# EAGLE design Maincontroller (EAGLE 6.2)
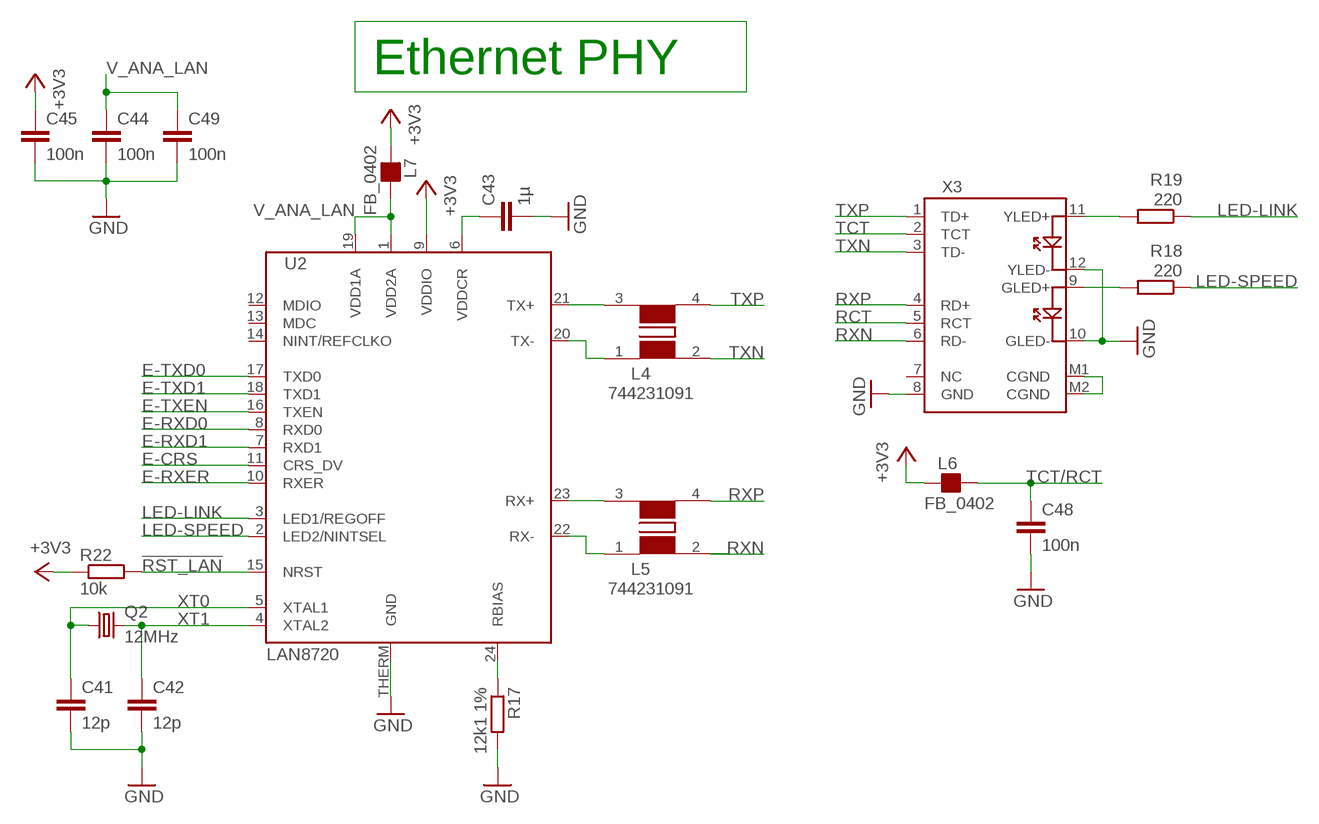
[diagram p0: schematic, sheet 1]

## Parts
C41  12p  C-EUC0402  [C0402]
C42  12p  C-EUC0402  [C0402]
C43  1µ  C-EUC0402  [C0402]
C44  100n  C-EUC0402  [C0402]
C45  100n  C-EUC0402  [C0402]
C48  100n  C-EUC0402  [C0402]
C49  100n  C-EUC0402  [C0402]
L4  744231091  WE-CNS_0805  [WE-CNS_0805]
L5  744231091  WE-CNS_0805  [WE-CNS_0805]
L6  FB_0402  [L0402]
L7  FB_0402  [L0402]
Q2  12MHz  CRYSTALHC49U-V  [HC49U-V]
R17  12k1 1%  R-EU_R0402  [R0402]
R18  220  R-EU_R0402  [R0402]
R19  220  R-EU_R0402  [R0402]
R22  10k  R-EU_R0402  [R0402]
U2  LAN8720  [QFN24_4MM]
X3  MAGJACK  [MAGJACK]

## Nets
!RST_LAN: R22.2 U2.15(NRST)
+3V3: C45.1 L6.1 L7.1 R22.1 U2.9(VDDIO)
E-CRS: U2.11(CRS_DV)
E-RXD0: U2.8(RXD0)
E-RXD1: U2.7(RXD1)
E-RXER: U2.10(RXER)
E-TXD0: U2.17(TXD0)
E-TXD1: U2.18(TXD1)
E-TXEN: U2.16(TXEN)
GND: C41.2 C42.2 C43.2 C44.2 C45.2 C48.2 C49.2 R17.2 U2.THERM(GND) X3.8(GND) X3.10(GLED-) X3.12(YLED-)
LED-LINK: R19.1 U2.3(LED1/REGOFF)
LED-SPEED: R18.1 U2.2(LED2/NINTSEL)
N$7: X3.M1(CGND) X3.M2(CGND)
N$9: C43.1 U2.6(VDDCR)
N$22: R19.2 X3.11(YLED+)
N$23: R18.2 X3.9(GLED+)
RBIAS: R17.1 U2.24(RBIAS)
RXN: L5.2 X3.6(RD-)
RXN-C: L5.1 U2.22(RX-)
RXP: L5.4 X3.4(RD+)
RXP-C: L5.3 U2.23(RX+)
TCT/RCT: C48.1 L6.2 X3.2(TCT) X3.5(RCT)
TXN: L4.2 X3.3(TD-)
TXN-C: L4.1 U2.20(TX-)
TXP: L4.4 X3.1(TD+)
TXP-C: L4.3 U2.21(TX+)
V_ANA_LAN: C44.1 C49.1 L7.2 U2.1(VDD2A) U2.19(VDD1A)
XT0: C41.1 Q2.1 U2.5(XTAL1)
XT1: C42.1 Q2.2 U2.4(XTAL2)
Unconnected: U2.12(MDIO) U2.13(MDC) U2.14(NINT/REFCLKO)

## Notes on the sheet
- Ethernet PHY
- TCT
- RCT

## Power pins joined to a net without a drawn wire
NC: X3.7(NC)

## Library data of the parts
C41-C45 C48 C49 = _rcl:C-EU: CAPACITOR, European symbol
L4 L5 = wuerth-elektronik:WE-CNS: SMD Multilayer Common-Mode Choke WE-CNS - Common mode data line filter - Fully shielded -- USB 2.0 -- IEEE 1394 -- Power supply systems -- Signal interfaces
L6 L7 = _rc-master-smd:FB_: FERRITE BEAD
Q2 = _crystal:CRYSTAL: CRYSTAL; OC_FARNELL: 1666969; OC_NEWARK: unknown
R17-R19 R22 = _rcl:R-EU_: RESISTOR, European symbol
U2 = _microbuilder:LAN8720: LAN8720A 10/100 Ethernet PHY Mouser: 886-LAN8720AI-CP
X3 = _IT-WNS:MAGJACK: MagJack von IT-WNS Art.Nr: RJ45-TRAFO-L AMPHENOL Connector FROM: "Drawing Nr. LMJ199 882X 110DTLX39J Datasheet: C:\Dokumente und Einstellungen\rene\Eigene Dateien\elektro\datenblätter\IT-WNS ArtNr RJ45-TRAFO-L.pdf

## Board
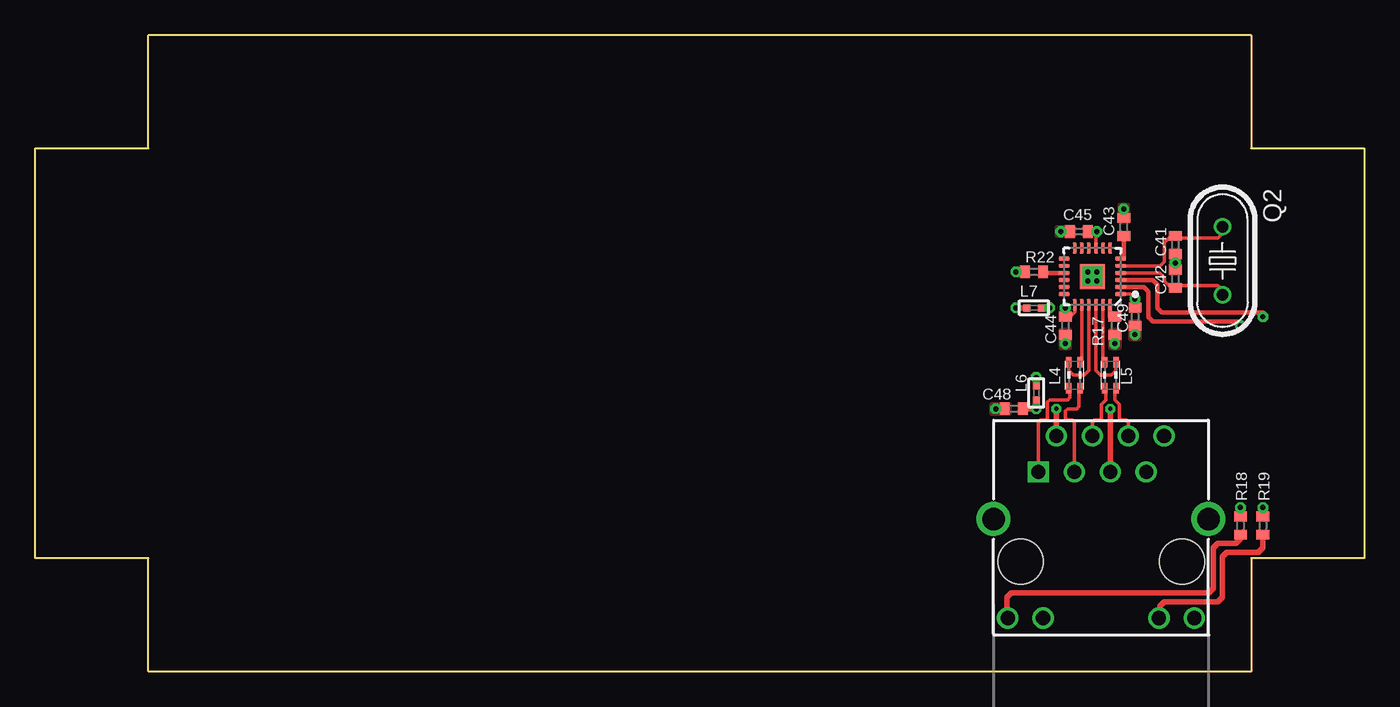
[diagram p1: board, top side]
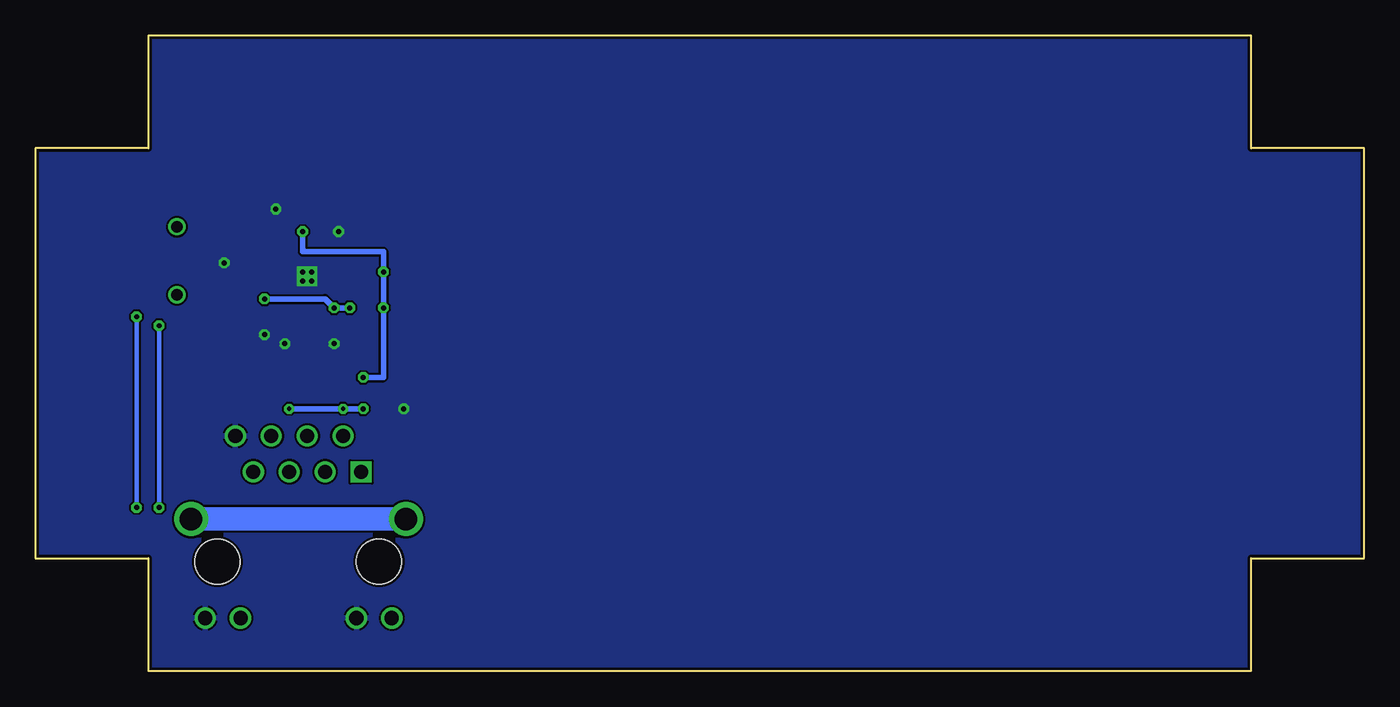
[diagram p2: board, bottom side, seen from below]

Size 94 x 45 mm. Coordinates in mm from the lower left corner, seen from the top.
Copper layers (1*16): Top 0.035mm / dielectric 1.5mm / Bottom 0.035mm
Design rules: minimum track width 0.15mm, minimum drill 0.3mm, track to track 0.15mm, track to pad 0.15mm, pad to pad 0.15mm, via to via 0.15mm, smd to smd 0mil, copper to edge 0.2mm, drill to drill 0.2mm, minimum pad ring 0.2mm, minimum via ring 0.2mm, stop-mask expansion 3mil, vias tented up to drill 0.8mm, thermal gap 0.15mm

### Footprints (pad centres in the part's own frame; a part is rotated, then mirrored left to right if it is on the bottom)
C0402 = smd 0.7 x 0.9: 1 -0.65,0; 2 0.65,0
WE-CNS_0805 = smd 0.75 x 0.4: 1 -0.925,0.4; 2 0.925,0.4; 3 -0.925,-0.4; 4 0.925,-0.4
L0402 = smd 0.5 x 0.5: 1 -0.508,0; 2 0.508,0
HC49U-V = drill 0.813: 1 -2.413,0; 2 2.413,0
R0402 = smd 0.7 x 0.9: 1 -0.65,0; 2 0.65,0
QFN24_4MM = smd 0.8 x 0.28: 1 -2,1.25; 2 -2,0.75; 3 -2,0.25; 4 -2,-0.25; 5 -2,-0.75; 6 -2,-1.25; 13 2,-1.25; 14 2,-0.75; 15 2,-0.25; 16 2,0.25; 17 2,0.75; 18 2,1.25 | smd 0.28 x 0.8: 7 -1.25,-2; 8 -0.75,-2; 9 -0.25,-2; 10 0.25,-2; 11 0.75,-2; 12 1.25,-2; 19 1.25,2; 20 0.75,2; 21 0.25,2; 22 -0.25,2; 23 -0.75,2; 24 -1.25,2 | smd 1.778 x 1.778: THERM 0,0
MAGJACK = drill 1 square: 1 3.175,17.445 | drill 1: 2 4.445,19.985; 3 5.715,17.445; 4 6.985,19.985; 5 8.255,17.445; 6 9.525,19.985; 7 10.795,17.445; 8 12.065,19.985; 9 1,7.1; 10 3.5,7.1; 11 11.7,7.1; 12 14.2,7.1 | drill 1.6: M1 0,14.1; M2 15.2,14.1 | hole 3.2: 1.905,11.095; 13.335,11.095

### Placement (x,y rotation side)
C41  80.64,30.16 270 top
C42  80.64,27.78 90 top
C43  76.99,31.43 90 top
C44  72.87,24.45 270 top
C45  73.82,31.11 180 top
C48  69.22,18.57 180 top
C49  77.79,25.08 270 top
L4  73.5,20.95 270 top
L5  76.04,20.95 270 top
L6  70.8,19.68 270 top
L7  70.64,25.72 0 top
Q2  83.98,29.05 270 top
R17  76.36,24.45 270 top
R18  85.25,10.32 270 top
R19  86.84,10.32 270 top
R22  70.64,28.26 0 top
U2  74.77,27.94 180 top
U$2  [KL_W_GEHÄUSE]  0,0 90 bottom
X3  67.79,-3.33 0 top

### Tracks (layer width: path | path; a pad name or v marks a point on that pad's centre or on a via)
!RST_LAN
  Top 0.305: U2.15 71.29,28.19 R22.2
+3V3  (via drill 0.35)
  Top 0.254: U2.9 75.02,31.11 v75.09,31.11 74.93,31.11
  Top 0.305: C45.1 74.93,31.11 75.02,31.11
  Top 0.406: L6.1 v70.8,20.8 | R22.1 v69.37,28.26 | L7.1 v69.37,25.72
  Bottom 0.406: v70.8,20.8 69.37,20.8 v69.37,25.72 v69.37,28.26 69.37,29.69 75.09,29.69 v75.09,31.11
GND  (via drill 0.35)
  Top 0.305: v75.09,27.62 U2.THERM 74.77,27.62
  other vias: 74.45,28.26 75.09,28.26 74.45,27.62 76.36,23.18 80.64,28.89 76.99,32.7 72.87,23.18 72.55,31.11 67.94,18.57 77.79,23.81
  pour Bottom: 0,45.09 93.98,45.09 93.98,0 0,0
  pour Top (no thermals): 76.68,24.13 76.04,24.13 76.04,22.86 76.68,22.86
  pour Top (no thermals): 76.68,31.75 77.31,31.75 77.31,33.02 76.68,33.02
  pour Top (no thermals): 73.18,24.13 72.55,24.13 72.55,22.86 73.18,22.86
  pour Top (no thermals): 73.5,30.8 73.5,31.43 72.23,31.43 72.23,30.8
  pour Top (no thermals): 67.63,18.89 67.63,18.26 68.9,18.26 68.9,18.89
  pour Top (no thermals): 80.33,28.1 80.96,28.1 80.96,29.84 80.33,29.84
  pour Top (no thermals): 78.11,24.77 77.47,24.77 77.47,23.5 78.11,23.5
LED-LINK  (via drill 0.35)
  Top 0.305: U2.3 79.06,27.69 79.38,27.37 79.38,25.72 79.69,25.4 86.84,25.4 v86.84,25.08 | v86.84,11.59 R19.1
  Bottom 0.305: v86.84,25.08 v86.84,11.59
LED-SPEED  (via drill 0.35)
  Top 0.305: U2.2 78.42,27.19 78.74,26.87 78.74,25.08 79.06,24.77 85.25,24.77 v85.25,24.45 | v85.25,11.59 R18.1
  Bottom 0.305: v85.25,24.45 v85.25,11.59
N$7
  Bottom 1.676: X3.M1 X3.M2
N$9
  Top 0.305: U2.6 76.99,29.19 C43.1
N$22
  Top 0.406: X3.11 79.53,3.77 79.53,4.6 79.85,4.92 83.66,4.92 83.98,5.24 83.98,8.1 84.3,8.41 86.52,8.41 86.84,8.73 R19.2
N$23
  Top 0.406: X3.9 68.74,3.77 68.74,5.24 69.06,5.56 83.03,5.56 83.34,5.87 83.34,8.73 83.66,9.05 84.93,9.05 85.25,9.37 R18.2
RBIAS
  Top 0.305: R17.1 76.02,25.08 U2.24
RXN
  Top 0.254: L5.2 76.36,20.03 76.36,19.21 76.68,18.89 76.68,17.94 76.83,17.78 77.17,17.78 77.33,17.62 77.33,16.65 X3.6
RXN-C
  Top 0.254: L5.1 76.44,21.27 76.12,20.95 75.34,20.95 75.02,21.27 U2.22
RXP
  Top 0.254: L5.4 75.72,20.03 75.72,19.21 75.41,18.89 75.41,17.94 75.25,17.78 74.92,17.78 74.76,17.62 74.76,16.65 X3.4
RXP-C
  Top 0.254: L5.3 75.52,21.88 U2.23
TCT/RCT  (via drill 0.3, 0.35)
  Top 0.406: L6.2 v70.8,18.57 C48.1 | 72.22,16.65 X3.2 v72.23,18.57 | 76.06,18.57 v76.04,18.57 X3.5 76.06,14.11
  Bottom 0.406: v76.04,18.57 v72.23,18.57 v70.8,18.57
TXN
  Top 0.254: 73.52,14.11 X3.3 73.5,17.62 73.34,17.78 73.03,17.78 72.87,17.94 72.87,18.41 73.03,18.57 73.66,18.57 73.82,18.73 73.82,20.03 L4.2
TXN-C
  Top 0.254: L4.1 74.02,21.88 U2.20
TXP
  Top 0.254: 70.95,14.11 X3.1 70.96,17.62 71.12,17.78 71.44,17.78 71.6,17.94 71.6,19.05 71.75,19.21 73.03,19.21 73.18,19.37 73.18,20.03 L4.4
TXP-C
  Top 0.254: L4.3 73.1,21.27 73.42,20.95 74.2,20.95 74.52,21.27 U2.21
V_ANA_LAN  (via drill 0.35)
  Top 0.254: 73.2,25.1 73.52,25.41 U2.19 | U2.1 77.47,26.69 77.79,26.37 v77.79,26.35 C49.1
  Top 0.305: C44.1 73.2,25.1
  Top 0.406: L7.2 v71.75,25.72 | C44.1 v72.87,25.72
  Bottom 0.406: v71.75,25.72 v72.87,25.72 73.5,26.35 v77.79,26.35
XT0
  Top 0.254: 80.64,30.64 83.66,30.65 83.98,30.97 Q2.1 | C41.1 80.64,30.64 | 80.64,30.64 80.63,30.65 80.17,30.65 79.85,30.34 79.85,29.01 79.53,28.69 U2.5
XT1
  Top 0.254: U2.4 79.53,28.19 79.85,27.87 79.85,27.61 80.17,27.29 80.64,27.29 C42.1 80.64,27.3 83.66,27.3 83.98,26.99 Q2.2

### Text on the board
tStop: Test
